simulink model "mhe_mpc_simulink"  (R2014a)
settings: Solver=ode45  StartTime=0.0  StopTime=100  RelTol=1e-3
libraries: simulink x1

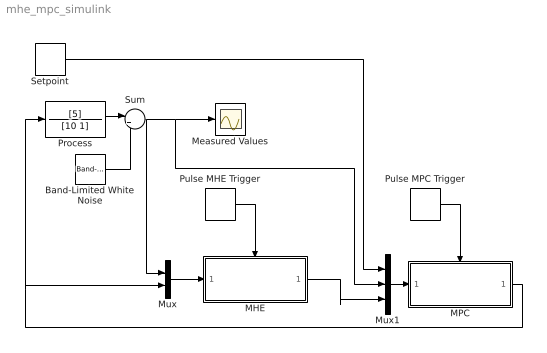
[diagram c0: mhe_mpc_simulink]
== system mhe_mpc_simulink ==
  Band-Limited White Noise : simulink/Sources/Band-Limited White Noise  Cov=[0.001]  Ts=1.0  seed=[23341]
  MHE : Subsystem  TreatAsAtomicUnit=on
  MPC : Subsystem  TreatAsAtomicUnit=on
  Measured Values : Scope
  Mux : Mux  Inputs=2
  Mux1 : Mux  Inputs=3
  Process : TransferFcn  Numerator=[5]  Denominator=[10 1]
  Pulse MHE Trigger : DiscretePulseGenerator  PulseType=Time based  Period=1  PulseWidth=5
  Pulse MPC Trigger : DiscretePulseGenerator  PulseType=Time based  Period=1  PulseWidth=5
  Setpoint : DiscretePulseGenerator  PulseType=Time based  Amplitude=10  Period=50  PulseWidth=30
  Sum : Sum  Inputs=|++
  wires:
  Process/1 -> Sum/1
  Band-Limited White Noise/1 -> Sum/2
  Sum/1 -> Mux/1, Mux1/2, Measured Values/1
  Mux/1 -> MHE/1(In1)
  Pulse MHE Trigger/1 -> MHE/Trigger
  MHE/1(Out1) -> Mux1/3
  Setpoint/1 -> Mux1/1
  Mux1/1 -> MPC/1(In1)
  MPC/1(Out1) -> Process/1, Mux/2
  Pulse MPC Trigger/1 -> MPC/Trigger

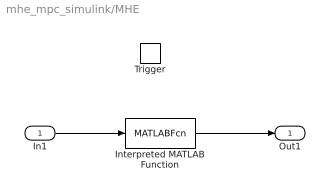
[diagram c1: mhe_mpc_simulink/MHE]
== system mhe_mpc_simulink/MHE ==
  In1 : Inport
  Trigger : TriggerPort
  Interpreted MATLAB Function : MATLABFcn  MATLABFcn=mhe  OutputDimensions=3
  Out1 : Outport  InitialOutput=[1 10 0]
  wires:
  In1/1 -> Interpreted MATLAB Function/1
  Interpreted MATLAB Function/1 -> Out1/1

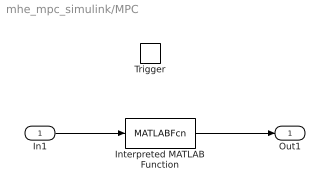
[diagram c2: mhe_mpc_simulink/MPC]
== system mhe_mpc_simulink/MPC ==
  In1 : Inport
  Trigger : TriggerPort
  Interpreted MATLAB Function : MATLABFcn  MATLABFcn=mpc  OutputDimensions=1
  Out1 : Outport  InitialOutput=[0]
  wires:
  In1/1 -> Interpreted MATLAB Function/1
  Interpreted MATLAB Function/1 -> Out1/1
